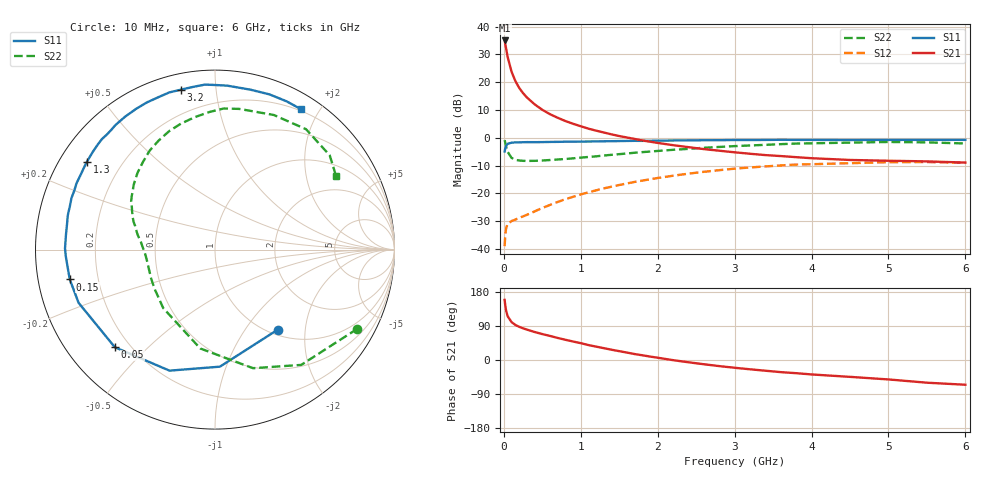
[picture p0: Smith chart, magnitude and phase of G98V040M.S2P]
! SIEMENS Small Signal Semiconductors
! BFG235
! Si NPN RF Bipolar Junction Transistor in SOT223
! VCE = 8 V  IC = 40 mA
! Common Emitter S-Parameters:  July  1994
# GHz  S  MA  R  50
!  f  S11  S21  S12  S22
! GHz  MAG  ANG  MAG  ANG  MAG  ANG  MAG  ANG
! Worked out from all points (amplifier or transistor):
!   40 points, 10 MHz to 6 GHz, reference 50 ohm
!   highest |S21| = 35.0 dB at 10 MHz (marker M1)
!   |S21| within 3 dB of that: start of sweep to 30.13 MHz
!   unconditionally stable (mu >= 1): 531.7 MHz to 1.267 GHz
!   at 200 MHz: K = 0.61, MSG = 23.4 dB, |S12| = -28.8 dB
!   at 1.5 GHz: K = 0.96, MSG = 8.8 dB, |S12| = -17.0 dB
!   at 6 GHz: K = 0.93, MSG = 0.1 dB, |S12| = -9.0 dB
!   S11 on the Smith chart (normalised r, x): 10 MHz: 1.09, -1.43; 50 MHz: 0.14, -0.40; 150 MHz: 0.10, -0.10; 1.3 GHz: 0.08, +0.31; 3.2 GHz: 0.08, +0.81; 6 GHz: 0.18, +1.77
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0.01  0.5666 -52.0  56.47 158.6  0.0112 70.2  0.9074 -29.1
0.02  0.6528 -87.6  47.87 141.9  0.0189 55.6  0.8021 -53.2
0.03  0.7205 -110.6  40.06 129.9  0.0235 46.1  0.694 -72.2
0.05  0.7793 -135.7  28.3 115.3  0.0284 34.0  0.5569 -98.5
0.1  0.8158 -158.7  15.49 100.0  0.0317 28.2  0.435 -131.6
0.15  0.826 -168.4  10.5 92.5  0.0337 29.9  0.4011 -147.2
0.2  0.8269 -173.3  7.887 87.6  0.0362 32.9  0.3902 -156.1
0.25  0.8322 -177.5  6.357 83.6  0.0385 36.0  0.3846 -161.9
0.3  0.8357 179.5  5.313 80.2  0.0411 38.9  0.3833 -166.3
0.4  0.8345 174.2  4.001 73.9  0.0473 43.5  0.3847 -172.1
0.5  0.8367 170.1  3.189 68.4  0.0545 47.0  0.3899 -176.4
0.6  0.8421 166.9  2.66 63.5  0.0619 49.0  0.398 -180.0
0.7  0.8445 162.9  2.291 58.2  0.07 50.8  0.4065 176.9
0.9  0.85 157.2  1.787 48.8  0.0866 51.3  0.4268 171.6
1.1  0.8569 150.7  1.459 39.4  0.1043 50.4  0.4517 166.2
1.3  0.8655 145.6  1.245 31.2  0.1229 48.7  0.4791 161.2
1.7  0.881 135.7  0.954 15.7  0.1606 42.3  0.5385 150.2
2.2  0.8942 124.0  0.736 -0.4  0.2075 32.2  0.6077 135.3
3.2  0.9112 101.9  0.516 -24.5  0.2921 8.2  0.7271 105.1
4.5  0.9127 77.6  0.399 -44.5  0.3489 -23.7  0.8184 66.4
5.5  0.9174 64.3  0.376 -59.9  0.3658 -46.4  0.8273 39.4
6  0.9174 58.5  0.358 -65.3  0.3538 -54.9  0.7896 31.4
